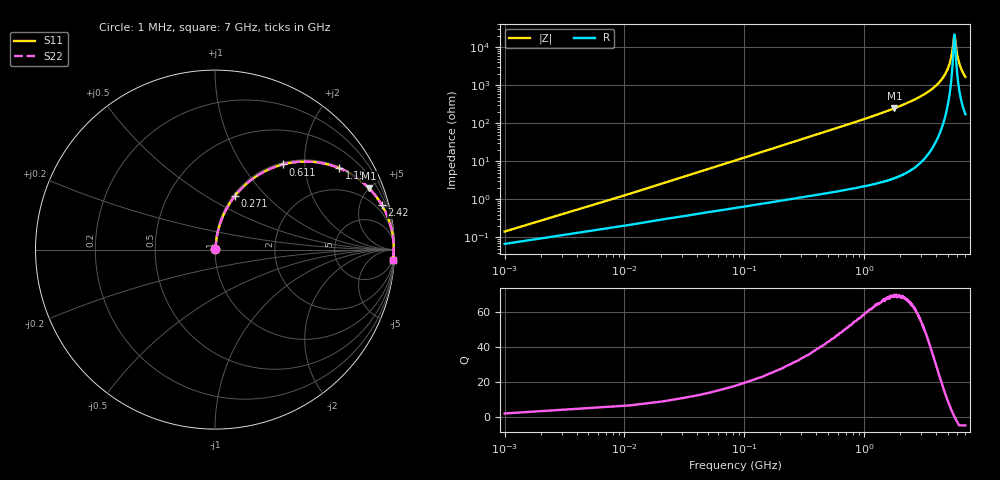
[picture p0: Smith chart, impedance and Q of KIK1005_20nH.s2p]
!version-3
!date-01.2023
!Series
# MHz S RI R 50
!Freq ReS11 ImS11 ReS21 ImS21 ReS12 ImS12 ReS22 ImS22
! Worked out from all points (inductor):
!   701 points, 1 MHz to 7 GHz, reference 50 ohm
!   read as one part in series: L = 20 nH near 31 MHz
!   highest Q = 69.3 at 1.79 GHz (marker M1), where L = 22.2 nH
!   self-resonance near 5.67 GHz
!   S11 on the Smith chart (normalised r, x): 1 MHz: 1.00, +0.00; 271 MHz: 1.02, +0.68; 611 MHz: 1.03, +1.55; 1.15 GHz: 1.05, +3.02; 2.42 GHz: 1.11, +7.44; 7 GHz: 4, -33
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1  0.000651 0.00126  0.9993 -0.00126  0.9993 -0.00126  0.000651 0.00126
41  0.00676 0.051  0.9932 -0.051  0.9932 -0.051  0.00676 0.051
71  0.0132 0.0876  0.9868 -0.0876  0.9868 -0.0876  0.0132 0.0876
151  0.0419 0.1805  0.9581 -0.1805  0.9581 -0.1805  0.0419 0.1805
271  0.1119 0.2999  0.8881 -0.2999  0.8881 -0.2999  0.1119 0.2999
611  0.3789 0.4746  0.6211 -0.4746  0.6211 -0.4746  0.3789 0.4746
1150  0.6919 0.4537  0.3081 -0.4537  0.3081 -0.4537  0.6919 0.4537
1170  0.6997 0.4504  0.3003 -0.4504  0.3003 -0.4504  0.6997 0.4504
1790  0.8585 0.3414  0.1415 -0.3414  0.1415 -0.3414  0.8585 0.3414
2340  0.923 0.2592  0.077 -0.2592  0.077 -0.2592  0.923 0.2592
2420  0.9293 0.2488  0.0707 -0.2488  0.0707 -0.2488  0.9293 0.2488
3510  0.9777 0.1362  0.0223 -0.1362  0.0223 -0.1362  0.9777 0.1362
4670  0.9933 0.0543  0.0067 -0.0543  0.0067 -0.0543  0.9933 0.0543
5010  0.9948 0.0346  0.00517 -0.0346  0.00517 -0.0346  0.9948 0.0346
5270  0.9954 0.0205  0.0046 -0.0205  0.0046 -0.0205  0.9954 0.0205
5440  0.9955 0.0117  0.00447 -0.0117  0.00447 -0.0117  0.9955 0.0117
5660  0.9955 0.000641  0.00455 -0.000641  0.00455 -0.000641  0.9955 0.000641
5720  0.9954 -0.00229  0.00461 0.00229  0.00461 0.00229  0.9954 -0.00229
5840  0.9952 -0.00805  0.0048 0.00805  0.0048 0.00805  0.9952 -0.00805
6020  0.9948 -0.0165  0.0052 0.0165  0.0052 0.0165  0.9948 -0.0165
6260  0.994 -0.0273  0.00596 0.0273  0.00596 0.0273  0.994 -0.0273
7000  0.9904 -0.0583  0.0096 0.0583  0.0096 0.0583  0.9904 -0.0583
